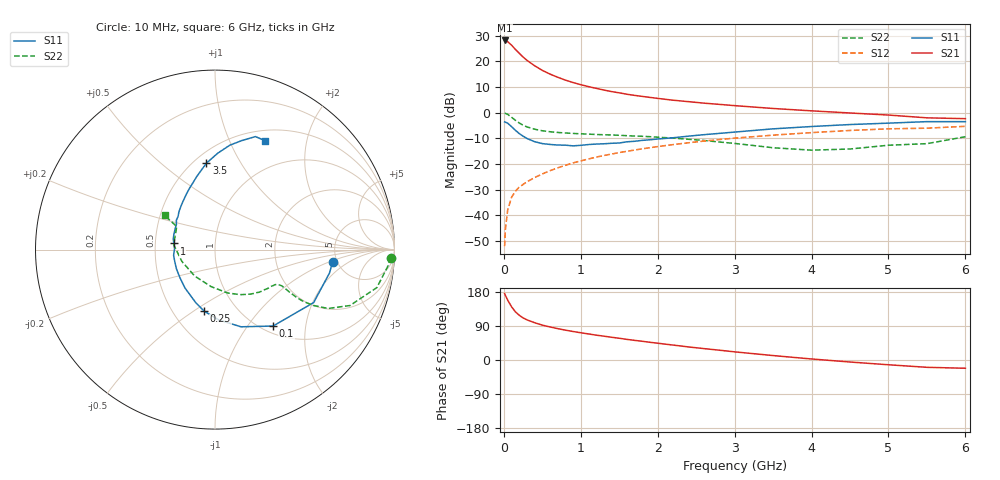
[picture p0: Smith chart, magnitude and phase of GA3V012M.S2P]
! Infineon Technologies  Discrete & RF Semiconductors
! BF775
! Si NPN RF Bipolar Junction Transistor in SOT23
! VCE = 3 V  IC = 12 mA
! Common Emitter S-Parameters:  May  1996
# GHz  S  MA  R  50
!  f  S11  S21  S12  S22
! GHz  MAG  ANG  MAG  ANG  MAG  ANG  MAG  ANG
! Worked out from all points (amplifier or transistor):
!   36 points, 10 MHz to 6 GHz, reference 50 ohm
!   highest |S21| = 28.1 dB at 10 MHz (marker M1)
!   |S21| within 3 dB of that: start of sweep to 135.1 MHz
!   unconditionally stable (mu >= 1): 496.5 MHz to 3.292 GHz
!   at 250 MHz: K = 0.74, MSG = 24.8 dB, |S12| = -28.0 dB
!   at 1.4 GHz: K = 1.12, MAG = 10.1 dB, |S12| = -16.1 dB
!   at 6 GHz: K = 0.95, MSG = 1.5 dB, |S12| = -5.3 dB
!   S11 on the Smith chart (normalised r, x): 10 MHz: 4.59, -1.10; 100 MHz: 1.12, -1.33; 250 MHz: 0.71, -0.55; 1 GHz: 0.63, +0.05; 3.5 GHz: 0.58, +0.72; 6 GHz: 0.62, +1.36
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0.01  0.6589 -5.9  25.55 175.3  0.0025 86.5  0.9791 -2.6
0.02  0.6512 -11.5  25.1 170.6  0.0053 87.7  0.9676 -5.5
0.05  0.624 -28.2  24.13 158.0  0.0127 76.9  0.9264 -13.2
0.1  0.5348 -52.8  20.71 140.5  0.0223 68.5  0.8141 -22.5
0.15  0.4538 -71.4  17.08 127.2  0.0294 64.3  0.7104 -27.5
0.2  0.392 -87.0  14.37 118.1  0.0354 63.5  0.6294 -29.6
0.25  0.3485 -99.9  12.16 111.1  0.0399 62.6  0.5695 -30.4
0.3  0.3143 -110.0  10.48 106.0  0.0449 63.2  0.5288 -30.4
0.4  0.2716 -128.0  8.212 98.4  0.0543 63.9  0.4765 -29.7
0.5  0.2498 -141.9  6.673 92.0  0.0639 65.0  0.4435 -28.9
0.6  0.2402 -153.1  5.651 87.2  0.074 65.7  0.4248 -28.5
0.7  0.2341 -163.4  4.903 82.8  0.084 66.0  0.4116 -28.7
0.8  0.2327 -172.3  4.312 78.8  0.0941 65.8  0.4018 -29.0
1  0.2309 171.5  3.511 71.9  0.1147 65.4  0.3876 -30.3
1.1  0.2393 166.4  3.221 68.8  0.1252 64.9  0.3814 -31.7
1.3  0.2475 155.2  2.762 62.9  0.1459 63.5  0.3709 -34.0
1.6  0.2705 142.7  2.288 54.4  0.1768 60.8  0.3558 -38.8
2.2  0.3241 123.1  1.749 39.4  0.2386 54.7  0.3197 -50.7
3.5  0.4837 95.7  1.207 11.7  0.3647 38.4  0.2072 -96.1
4.5  0.5869 82.0  0.986 -5.3  0.4499 25.1  0.1958 -160.3
5.5  0.6688 70.3  0.793 -19.3  0.4982 10.4  0.2489 148.9
6  0.6679 65.4  0.764 -21.8  0.542 6.3  0.3396 145.9
